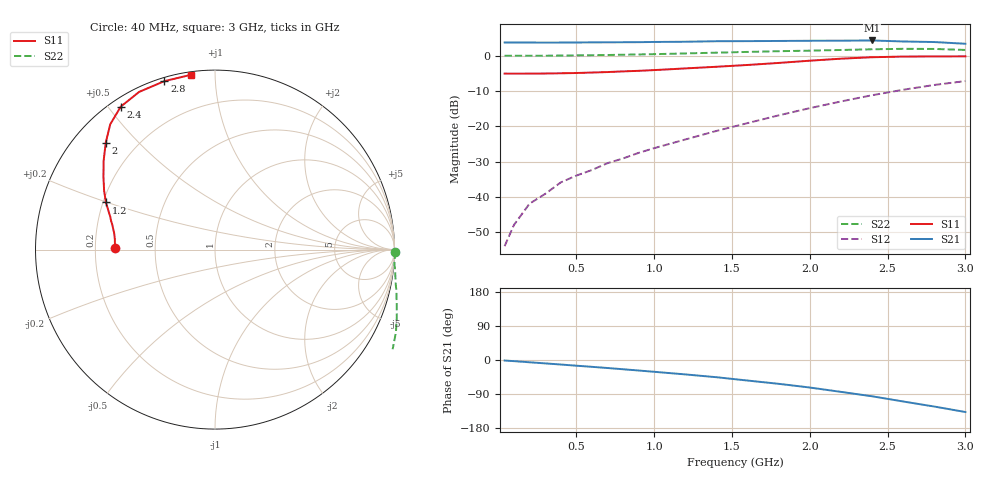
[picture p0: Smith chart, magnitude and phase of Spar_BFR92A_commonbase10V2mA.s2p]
! Filename:  BFR92ACF.S2P  Version:  2.0
! NXP part #: BFR92A  Date: Jul 1990
! Bias condition: Vce=10V, Ic=2mA
! COMMON BASE
#  MHz  S  MA  R  50
! Freq  S11  S21  S12  S22
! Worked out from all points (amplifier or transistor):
!   21 points, 40 MHz to 3 GHz, reference 50 ohm
!   highest |S21| = 4.3 dB at 2.4 GHz (marker M1)
!   |S21| within 3 dB of that: start of sweep to end of sweep
!   unconditionally stable (mu >= 1): nowhere
!   at 300 MHz: K = -0.22, MSG = 21.5 dB, |S12| = -39.2 dB
!   at 1 GHz: K = -0.79, MSG = 15.1 dB, |S12| = -26.2 dB
!   at 3 GHz: K = -0.47, MSG = 5.3 dB, |S12| = -7.2 dB
!   S11 on the Smith chart (normalised r, x): 40 MHz: 0.28, +0.01; 1.2 GHz: 0.21, +0.20; 2 GHz: 0.09, +0.41; 2.4 GHz: 0.03, +0.54; 2.8 GHz: 0.02, +0.74; 3 GHz: 0.02, +0.87
40  0.559 179.0  1.546 -1.4  0.002 74.5  1.002 -0.7
100  0.558 177.9  1.543 -3.0  0.004 87.0  1.004 -1.4
200  0.559 176.0  1.542 -6.0  0.008 93.8  1.003 -3.1
300  0.561 174.1  1.539 -8.9  0.011 99.0  1.003 -4.7
400  0.565 172.3  1.541 -11.9  0.016 103.0  1.009 -6.2
500  0.57 170.5  1.543 -15.0  0.02 106.1  1.014 -7.8
600  0.579 168.5  1.551 -18.0  0.024 109.7  1.019 -9.4
700  0.588 166.5  1.553 -21.1  0.03 112.9  1.026 -11.0
800  0.601 164.5  1.557 -24.4  0.035 115.4  1.036 -12.7
900  0.612 162.5  1.56 -27.7  0.042 118.2  1.045 -14.6
1000  0.627 160.6  1.571 -31.1  0.049 120.5  1.055 -16.3
1200  0.662 156.6  1.582 -38.0  0.065 124.5  1.08 -20.3
1400  0.699 152.1  1.609 -45.4  0.086 126.6  1.108 -24.5
1600  0.741 147.0  1.614 -54.2  0.111 128.3  1.135 -29.3
1800  0.792 141.6  1.623 -62.8  0.143 127.9  1.162 -34.8
2000  0.852 135.6  1.633 -72.6  0.181 126.4  1.183 -41.3
2200  0.91 129.9  1.637 -84.1  0.225 123.7  1.209 -48.9
2400  0.954 123.4  1.65 -95.7  0.276 119.8  1.236 -57.3
2600  0.975 115.7  1.596 -109.5  0.33 115.2  1.256 -65.7
2800  0.98 106.7  1.567 -122.8  0.386 109.4  1.251 -73.9
3000  0.983 97.8  1.481 -137.3  0.438 103.8  1.21 -82.4
